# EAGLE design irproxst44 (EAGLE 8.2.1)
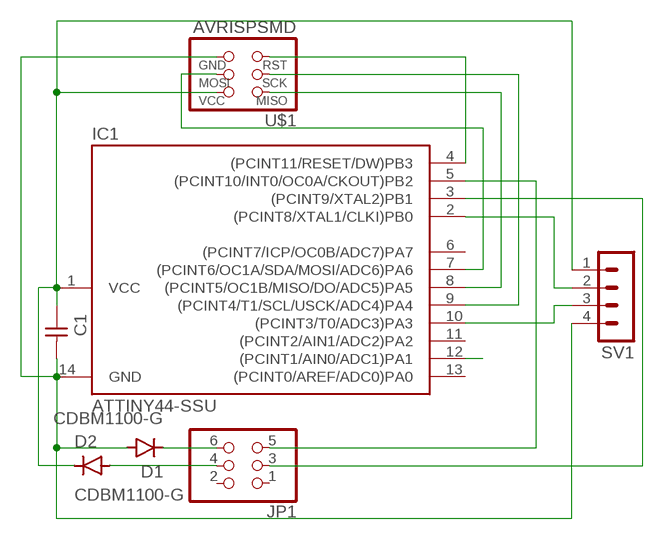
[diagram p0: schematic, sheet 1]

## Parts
C1  CAP-UNPOLARIZEDFAB  [C1206FAB]
D1  CDBM1100-G  [MINI-SMA]
D2  CDBM1100-G  [MINI-SMA]
IC1  ATTINY44-SSU  [SOIC14]
JP1  PINHD-2X3-SMD  [2X03SMD]
SV1  MA04-1  [MA04-1]
U$1  AVRISPSMD  [2X03SMD]

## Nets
N$1: IC1.4((PCINT11/RESET/DW)PB3) U$1.5(RST)
N$2: IC1.8((PCINT5/OC1B/MISO/DO/ADC5)PA5) U$1.1(MISO)
N$3: IC1.7((PCINT6/OC1A/SDA/MOSI/ADC6)PA6) U$1.4(MOSI)
N$4: IC1.9((PCINT4/T1/SCL/USCK/ADC4)PA4) U$1.3(SCK)
N$5: C1.1 D2.KATHODE IC1.1(VCC) SV1.1 U$1.2(VCC)
N$6: C1.2 D1.ANODE IC1.14(GND) SV1.4 U$1.6(GND)
N$7: IC1.5((PCINT10/INT0/OC0A/CKOUT)PB2) JP1.5
N$8: IC1.12((PCINT1/AIN0/ADC1)PA1)
N$9: IC1.2((PCINT8/XTAL1/CLKI)PB0) SV1.2
N$10: IC1.10((PCINT3/T0/ADC3)PA3) SV1.3
N$11: IC1.3((PCINT9/XTAL2)PB1) JP1.3
N$12: D1.KATHODE JP1.6
N$13: D2.ANODE JP1.4
Unconnected: IC1.6((PCINT7/ICP/OC0B/ADC7)PA7) IC1.11((PCINT2/AIN1/ADC2)PA2) IC1.13((PCINT0/AREF/ADC0)PA0) JP1.1 JP1.2

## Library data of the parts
C1 = fab:CAP-UNPOLARIZED
D1 D2 = fab:CDBM1100-G: Diode schottky 100V 1A mini-SMA as found in the fablab inventory
IC1 = fab:ATTINY44
JP1 = fab:PINHD-2X3-SMD: PIN HEADER
SV1 = con-lstb:MA04-1: PIN HEADER; OC_FARNELL: unknown; OC_NEWARK: unknown
U$1 = fab:AVRISP

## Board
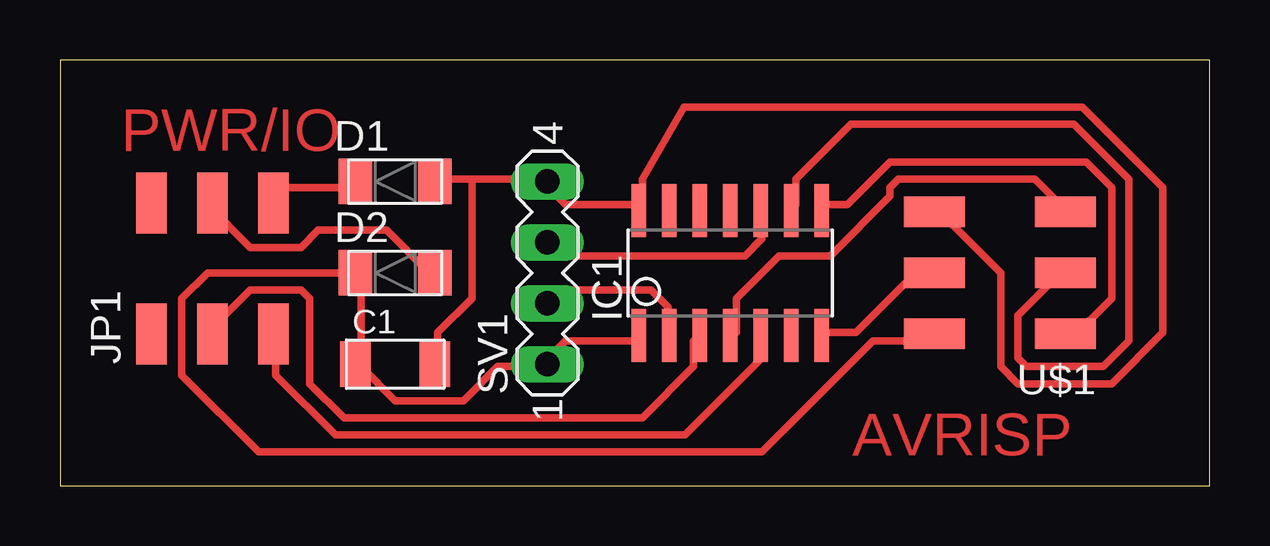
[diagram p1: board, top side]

Size 47.93 x 17.77 mm. Coordinates in mm from the lower left corner, seen from the top.
Outline: 0,0 47.93,0 47.93,17.77 0,17.77 0,0
Copper layers (1*16): Top 0.035mm / dielectric 1.5mm / Bottom 0.035mm
Design rules "default *": minimum track width 12mil, minimum drill 0.35mm, track to track 16mil, track to pad 16mil, pad to pad 16mil, via to via 16mil, smd to smd 16mil, copper to edge 40mil, drill to drill 6mil, minimum pad ring 10mil, minimum via ring 8mil, stop-mask expansion 4mil, vias tented up to drill 0mil, thermal gap 10mil

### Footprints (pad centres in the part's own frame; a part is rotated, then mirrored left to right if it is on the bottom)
C1206FAB = smd 1.27 x 1.905: 1 -1.651,0; 2 1.651,0
MINI-SMA = smd 1.4 x 1.9: ANODE 1.65,0; KATHODE -1.65,0
SOIC14 = smd 0.61 x 2.21: 1 -3.81,-2.603; 2 -2.54,-2.603; 3 -1.27,-2.603; 4 0,-2.603; 5 1.27,-2.603; 6 2.54,-2.603; 7 3.81,-2.603; 8 3.81,2.603; 9 2.54,2.603; 10 1.27,2.603; 11 0,2.603; 12 -1.27,2.603; 13 -2.54,2.603; 14 -3.81,2.603
2X03SMD = smd 2.54 x 1.27: 1 -2.54,2.54; 2 2.92,2.54; 3 -2.54,0; 4 2.92,0; 5 -2.54,-2.54; 6 2.92,-2.54
MA04-1 = drill 1.016 long: 1 -3.81,0; 2 -1.27,0; 3 1.27,0; 4 3.81,0

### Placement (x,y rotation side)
C1  13.97,5.08 0 top
D1  13.97,12.7 0 top
D2  13.97,8.89 0 top
IC1  27.94,8.89 0 top
JP1  6.35,8.89 90 top
SV1  20.32,8.89 90 top
U$1  39.37,8.89 180 top

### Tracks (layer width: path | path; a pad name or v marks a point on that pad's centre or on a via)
N$1
  Top 0.305: IC1.4 28.19,6.4 28.19,7.82 29.97,9.6 32.11,9.6 34.59,12.09 34.59,12.45 34.95,12.8 40.64,12.8 41.71,11.73 U$1.5
N$2
  Top 0.305: IC1.8 31.75,11.73 32.82,11.73 34.59,13.51 42.77,13.51 43.84,12.45 43.84,7.82 42.06,6.04 U$1.1
N$3
  Top 0.305: U$1.4 35.66,8.89 33.17,6.4 31.75,6.4 IC1.7
N$4
  Top 0.305: IC1.9 30.68,11.73 30.68,12.8 32.97,15.09 42.27,15.09 44.55,12.8 44.55,6.04 43.48,4.98 40.28,4.98 39.93,5.33 39.93,7.11 41.71,8.89 U$1.3
N$5
  Top 0.305: IC1.1 23.93,6.04 21.08,6.04 20.37,5.33 SV1.1 20.02,4.98 18.24,4.98 16.82,3.56 13.97,3.56 12.55,4.98 C1.1 12.55,5.33 12.55,8.89 D2.KATHODE 6.15,8.89 5.08,7.82 5.08,4.62 8.28,1.42 29.26,1.42 33.88,6.04 36.37,6.04 U$1.2
N$6
  Top 0.305: 17.17,12.8 20.02,12.8 SV1.4 20.37,12.45 21.08,11.73 23.93,11.73 IC1.14 24.28,11.73 24.28,12.8 26.01,15.8 42.62,15.8 45.97,12.45 45.97,6.4 43.84,4.27 39.93,4.27 39.22,4.98 39.22,8.89 36.73,11.38 U$1.6 | 17.17,12.8 15.75,12.8 D1.ANODE | 17.17,12.8 17.17,7.82 15.75,6.4 15.75,5.33 C1.2
N$7
  Top 0.305: IC1.5 29.26,6.04 29.26,5.33 26.06,2.13 11.48,2.13 8.99,4.62 8.99,6.04 JP1.5
N$9
  Top 0.305: IC1.2 25.35,6.4 25.35,7.47 24.64,8.18 20.73,8.18 20.37,7.82 SV1.2
N$10
  Top 0.305: IC1.10 29.26,11.38 29.26,10.31 28.55,9.6 20.73,9.6 20.37,9.96 SV1.3
N$11
  Top 0.305: IC1.3 26.42,6.04 26.42,4.98 24.28,2.85 11.84,2.85 10.41,4.27 10.41,7.82 10.06,8.18 7.92,8.18 6.15,6.4 JP1.3
N$12
  Top 0.305: D1.KATHODE 12.19,12.45 9.35,12.45 8.99,12.09 JP1.6
N$13
  Top 0.305: D2.ANODE 15.39,8.89 13.61,10.67 10.77,10.67 10.06,9.96 7.92,9.96 6.15,11.73 JP1.4

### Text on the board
Top: PWR/IO | AVRISP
